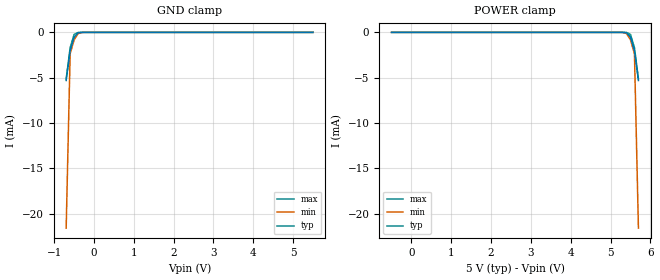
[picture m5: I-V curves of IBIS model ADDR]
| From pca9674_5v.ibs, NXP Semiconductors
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[Model]   ADDR
Model_type Input
Vinh=3.5
Vinl=1.5
C_comp   1.7p   1.5p   1.9p
[Model Spec]
Vinh   2.31   1.61   3.85
Vinl   0.99   0.69   1.65
[Temperature Range] 27   85   -40
[Voltage Range]   5   4.5   5.5
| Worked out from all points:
|   GND clamp passes 1 mA (typ) near -0.53 V on its own axis
[GND Clamp]
-700mV    -5.302mA   -21.58mA   -5.122mA
-600mV    -2.04mA    -2.358mA   -1.687mA
-500mV    -525.2uA   -816.9uA   -228.9uA
-400mV    -48.21uA   -135uA     -7.763uA
-200mV    -27.28nA   -200nA     -811.9pA
5.5V      106.9pA    399pA      72.28pA
[POWER Clamp]
-500mV    106.9pA    399pA      72.28pA
5.2V      -27.28nA   -200nA     -811.9pA
5.4V      -48.21uA   -135uA     -7.763uA
5.5V      -525.2uA   -816.9uA   -228.9uA
5.6V      -2.04mA    -2.358mA   -1.687mA
5.7V      -5.302mA   -21.58mA   -5.122mA
